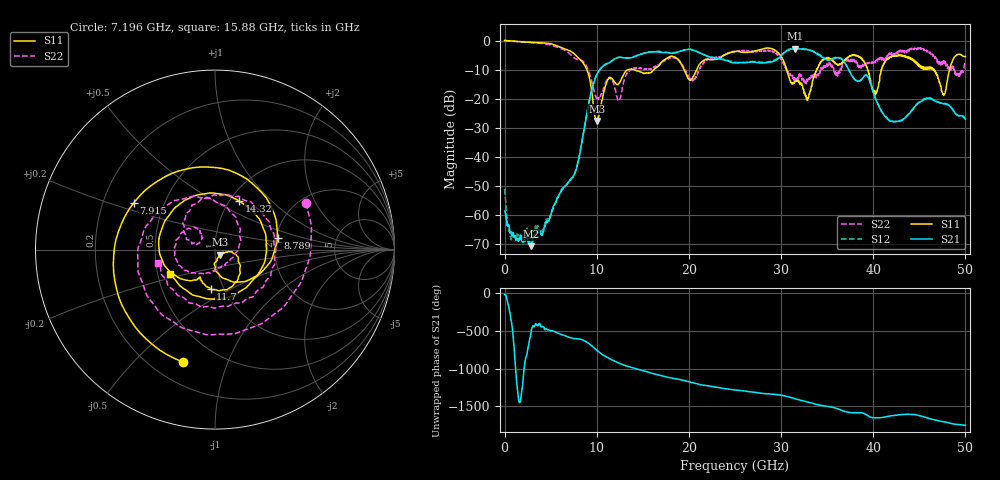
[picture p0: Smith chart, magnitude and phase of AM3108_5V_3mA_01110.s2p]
# Hz S DB R 50.0
!freq dBS11 angS11 dBS21 angS21 dBS12 angS12 dBS22 angS22
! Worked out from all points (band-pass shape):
!   1601 points, 10 MHz to 50 GHz, reference 50 ohm
!   highest |S21| = -2.76 dB at 31.53 GHz (marker M1); lowest = -70.7 dB at 2.884 GHz (marker M2)
!   |S21| within 3 dB of the highest: 13.94 GHz to 22.47 GHz (8.533 GHz wide, 46.9 % of centre); 29.85 GHz to 34.47 GHz (4.617 GHz wide, 14.4 % of centre)
!   lowest |S11| = -27.6 dB at 10.01 GHz (marker M3), VSWR 1.09, Z = 53 - j3.05 ohm
!   |S11| at or under -10 dB: 8.937 GHz to 13.38 GHz (4.448 GHz wide, 39.9 % of centre); 14.08 GHz to 16.21 GHz (2.13 GHz wide, 14.1 % of centre); 30.62 GHz to 33.85 GHz (3.229 GHz wide, 10 % of centre)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
!   |S22| runs from -20.8 to 0.0 dB; largest |S21 - S12| = 0.024
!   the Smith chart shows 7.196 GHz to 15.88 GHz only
!   S11 on the Smith chart (normalised r, x): 7.196 GHz: 0.32, -0.70; 7.915 GHz: 0.33, +0.24; 8.789 GHz: 2.04, +0.31; 11.7 GHz: 0.87, -0.40; 14.32 GHz: 1.10, +0.66; 15.88 GHz: 0.58, -0.17
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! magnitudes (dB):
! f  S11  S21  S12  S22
! 10 MHz  0.0  -58.6  -51.1  0.0
! 697.4 MHz  -0.1  -65.7  -67.9  -0.2
! 2.884 GHz  -0.6  -70.7  -69.6  -0.7
! 7.196 GHz  -3.7  -47.6  -48.0  -4.9
! 7.915 GHz  -5.7  -42.5  -42.6  -6.4
! 8.352 GHz  -6.9  -35.7  -35.6  -6.8
! 8.789 GHz  -9.0  -27.6  -27.5  -8.2
! 10.01 GHz  -27.6  -11.8  -11.7  -19.6
! 11.7 GHz  -13.2  -6.9  -6.8  -13.6
! 14.32 GHz  -10.4  -5.3  -5.1  -9.6
! 15.88 GHz  -11.0  -3.9  -3.8  -9.8
! 16.69 GHz  -8.7  -3.9  -3.6  -8.5
! 20.41 GHz  -12.6  -3.2  -3.1  -13.9
! 25 GHz  -3.8  -7.7  -7.5  -3.8
! 29.16 GHz  -3.0  -7.2  -6.9  -3.7
! 31.53 GHz  -14.1  -2.8  -2.7  -13.8
! 33.35 GHz  -15.5  -3.6  -3.4  -12.7
! 38 GHz  -4.9  -13.4  -13.4  -6.6
! 40.22 GHz  -18.7  -19.8  -19.7  -7.6
! 41.69 GHz  -6.0  -27.4  -27.1  -5.2
! 47.66 GHz  -18.9  -21.7  -21.6  -7.7
! 50 GHz  -5.5  -26.9  -26.6  -6.9
